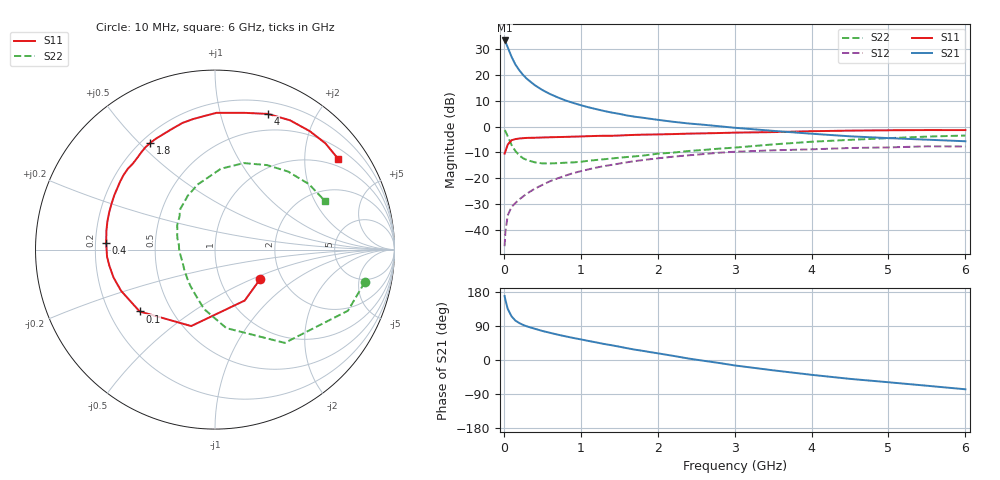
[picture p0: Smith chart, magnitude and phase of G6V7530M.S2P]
! SIEMENS Small Signal Semiconductors
! BFG193
! Si NPN RF Bipolar Junction Transistor in SOT223
! VCE = 0.75 V  IC = 30 mA
! Common Emitter S-Parameters:  August  1996
# GHz  S  MA  R  50
!  f  S11  S21  S12  S22
! GHz  MAG  ANG  MAG  ANG  MAG  ANG  MAG  ANG
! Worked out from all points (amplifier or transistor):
!   36 points, 10 MHz to 6 GHz, reference 50 ohm
!   highest |S21| = 33.2 dB at 10 MHz (marker M1)
!   |S21| within 3 dB of that: start of sweep to 55.4 MHz
!   unconditionally stable (mu >= 1): 384.5 MHz to 4.285 GHz
!   at 250 MHz: K = 0.89, MSG = 23.5 dB, |S12| = -27.0 dB
!   at 1.4 GHz: K = 1.10, MAG = 8.2 dB, |S12| = -14.8 dB
!   at 6 GHz: K = 1.00, MSG = 1.0 dB, |S12| = -7.7 dB
!   S11 on the Smith chart (normalised r, x): 10 MHz: 1.56, -0.55; 100 MHz: 0.33, -0.32; 400 MHz: 0.24, +0.03; 1.8 GHz: 0.23, +0.54; 4 GHz: 0.32, +1.41; 6 GHz: 0.77, +2.85
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0.01  0.3004 -32.6  45.81 168.7  0.0049 83.3  0.854 -12.3
0.02  0.3286 -59.7  43.53 158.9  0.0091 73.5  0.8152 -24.7
0.05  0.4462 -107.3  33.96 135.1  0.0192 59.8  0.6491 -53.2
0.1  0.5432 -140.6  22.19 115.3  0.028 54.1  0.4418 -81.8
0.15  0.5714 -156.3  15.73 104.0  0.0333 53.0  0.3362 -100.5
0.2  0.5866 -164.7  12.23 97.6  0.0391 54.9  0.278 -112.4
0.25  0.5955 -171.4  9.896 92.6  0.0446 56.5  0.2441 -124.2
0.3  0.6028 -176.2  8.31 88.7  0.0507 57.8  0.2257 -132.5
0.4  0.6071 176.7  6.313 82.6  0.0628 59.6  0.2038 -147.4
0.5  0.6139 170.4  5.068 76.7  0.0746 59.4  0.1942 -158.3
0.6  0.6199 165.2  4.24 71.8  0.0878 58.9  0.1935 -166.4
0.7  0.6252 160.5  3.65 66.9  0.1001 57.6  0.1963 -173.9
0.9  0.6375 151.7  2.858 58.3  0.1258 54.2  0.2027 172.9
1.1  0.6503 144.4  2.35 50.3  0.1488 50.5  0.2179 163.7
1.4  0.6625 133.7  1.861 39.0  0.1816 43.7  0.2415 150.5
1.8  0.6956 121.2  1.481 24.4  0.2242 34.5  0.2738 135.9
2.2  0.7139 109.6  1.234 11.0  0.2614 24.3  0.3131 123.7
3.5  0.7796 77.8  0.824 -27.2  0.3472 -8.2  0.4515 85.9
4  0.8114 68.7  0.726 -39.1  0.3627 -17.7  0.508 71.6
4.5  0.8331 59.8  0.647 -49.8  0.3846 -27.4  0.5528 58.4
5.5  0.8539 43.9  0.557 -67.9  0.4143 -49.4  0.6379 34.9
6  0.8523 36.4  0.519 -77.3  0.4124 -61.8  0.6704 23.7
